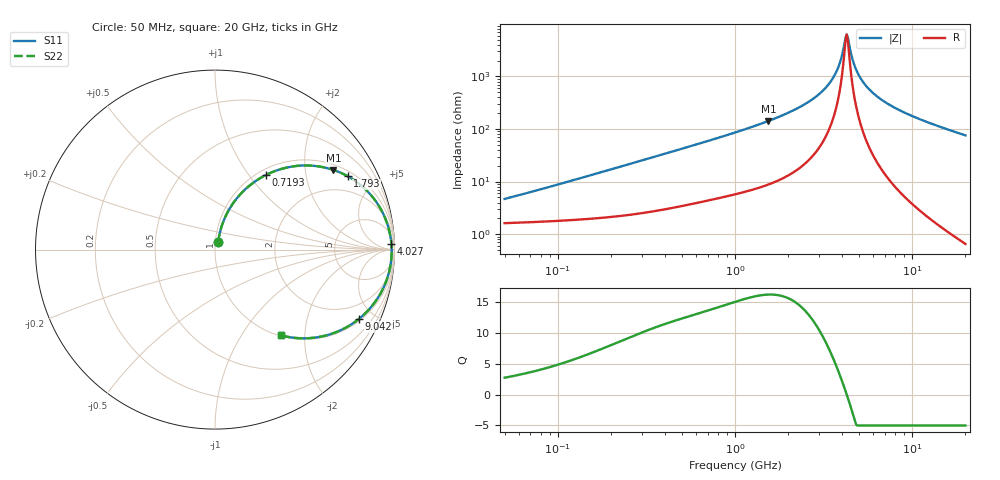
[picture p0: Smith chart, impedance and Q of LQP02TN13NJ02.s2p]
!Murata Part Number: LQP02TN13NJ02
!These Parameters are Measured in Series Mode Connection
!  o--[Z]--o
!Port1  Port2
!  o-------o
!Freq. Start=50[MHz] Stop=20[GHz], 401[Steps]
# Hz S RI R 50
!Freq.(Hz) S11(Real) S11(Imag) S21(Real) S21(Imag) S12(Real) S12(Imag) S22(Real) S22(Imag)
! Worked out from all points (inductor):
!   401 points, 50 MHz to 20 GHz, reference 50 ohm
!   read as one part in series: L = 13.8 nH near 56.37 MHz
!   highest Q = 16.1 at 1.544 GHz (marker M1), where L = 14.6 nH
!   self-resonance near 4.212 GHz
!   S11 on the Smith chart (normalised r, x): 50 MHz: 1.03, +0.09; 719.3 MHz: 1.09, +1.21; 1.793 GHz: 1.22, +3.47; 4.027 GHz: 23, +47; 9.042 GHz: 1.10, -4.12; 20 GHz: 1.01, -1.52
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5e7  0.0177 0.0424  0.9823 -0.0424  0.9823 -0.0424  0.0177 0.0424
1.364002e8  0.0314 0.1109  0.9686 -0.1109  0.9686 -0.1109  0.0314 0.1109
3.721004e8  0.11 0.2709  0.89 -0.2709  0.89 -0.2709  0.11 0.2709
7.192613e8  0.283 0.4153  0.717 -0.4153  0.717 -0.4153  0.283 0.4153
1e9  0.4282 0.4625  0.5718 -0.4625  0.5718 -0.4625  0.4282 0.4625
1.544007e9  0.66 0.4438  0.34 -0.4438  0.34 -0.4438  0.66 0.4438
1.793498e9  0.7386 0.4092  0.2614 -0.4092  0.2614 -0.4092  0.7386 0.4092
2.728004e9  0.9131 0.2435  0.0869 -0.2435  0.0869 -0.2435  0.9131 0.2435
3.168813e9  0.9516 0.1666  0.0484 -0.1666  0.0484 -0.1666  0.9516 0.1666
3.519108e9  0.9699 0.1095  0.0301 -0.1095  0.0301 -0.1095  0.9699 0.1095
3.792786e9  0.9785 0.0677  0.0215 -0.0677  0.0215 -0.0677  0.9785 0.0677
4.026975e9  0.9827 0.0338  0.0173 -0.0338  0.0173 -0.0338  0.9827 0.0338
4.149438e9  0.9838 0.0167  0.0162 -0.0167  0.0162 -0.0167  0.9838 0.0167
4.275624e9  0.9844 -0.000402  0.0156 0.000402  0.0156 0.000402  0.9844 -0.000402
4.405649e9  0.9843 -0.0175  0.0157 0.0175  0.0157 0.0175  0.9843 -0.0175
4.748272e9  0.9815 -0.0603  0.0185 0.0603  0.0185 0.0603  0.9815 -0.0603
5.194772e9  0.9731 -0.1113  0.0269 0.1113  0.0269 0.1113  0.9731 -0.1113
6.034176e9  0.9469 -0.1941  0.0531 0.1941  0.0531 0.1941  0.9469 -0.1941
7.442007e9  0.885 -0.3011  0.115 0.3011  0.115 0.3011  0.885 -0.3011
9.041845e9  0.8034 -0.3851  0.1966 0.3851  0.1966 0.3851  0.8034 -0.3851
1.334722e10  0.5921 -0.4845  0.4079 0.4845  0.4079 0.4845  0.5921 -0.4845
2e10  0.3661 -0.4774  0.6339 0.4774  0.6339 0.4774  0.3661 -0.4774
